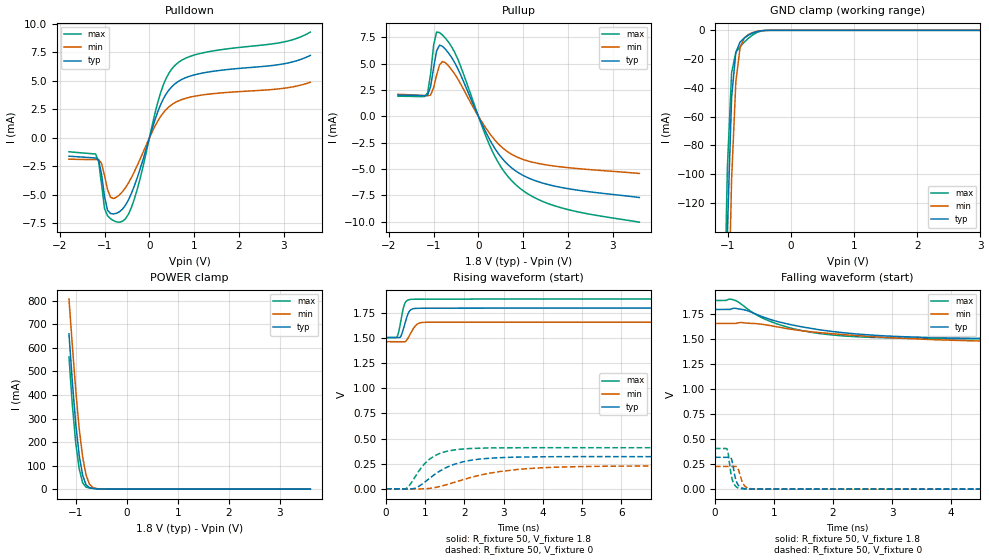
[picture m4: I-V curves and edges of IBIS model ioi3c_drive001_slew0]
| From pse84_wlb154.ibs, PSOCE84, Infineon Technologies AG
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[Model] ioi3c_drive001_slew0
Model_type I/O
Enable   Active-High
Vinl  =  0.54
Vinh  =  1.26
Vmeas =  0.9
Cref  =  15e-12
| Capacitance   typ   min   max
C_comp   9.12545e-13 8.87504e-13 9.42456e-13
| Variables   typ   min   max
[GND Clamp Reference]   0   0   0
[POWER Clamp Reference]   1.8   1.66   1.89
[Pulldown Reference]   0   0   0
[Pullup Reference]   1.8   1.66   1.89
[Temperature Range]   25   125   -40
[Voltage Range]   1.8   1.66   1.89
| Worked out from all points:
|   slope of the pulldown table from 0 to 0.27 V, typ, clamps not added: 87.9 ohm
|   slope of the pullup table from 0 to 0.27 V, typ, clamps not added: 115 ohm
|   GND clamp passes 1 mA (typ) near -0.55 V on its own axis
|   POWER clamp passes 1 mA (typ) near -0.54 V on its own axis
|   falling waveform, R_fixture 50, V_fixture 1.8: 20-80 % time 1.48ns typ, 2.34ns min, 990ps max; typ from 1.8 V to 1.51 V
|   falling waveform, R_fixture 50, V_fixture 0: 20-80 % time 73ps typ, 80.4ps min, 68.9ps max; typ from 0.319 V to 0 V
|   rising waveform, R_fixture 50, V_fixture 1.8: 20-80 % time 136ps typ, 178ps min, 116ps max; typ from 1.51 V to 1.8 V
|   rising waveform, R_fixture 50, V_fixture 0: 20-80 % time 866ps typ, 1.54ns min, 553ps max; typ from 0 V to 0.319 V
[GND Clamp]
| Voltage   I(typ)   I(min)   I(max)
-1.204V   -737.9mA   -831.5mA   -678.7mA
-1.07V    -303.2mA   -410.8mA   -239.8mA
-1.003V   -139.9mA   -232.2mA   -95.74mA
-936.6mV  -46.51mA   -103.5mA   -29.5mA
-869.7mV  -15.31mA   -35.88mA   -15.36mA
-802.8mV  -8.166mA   -12.13mA   -11.29mA
-735.9mV  -5.335mA   -5.292mA   -8.195mA
-669mV    -3.356mA   -2.85mA    -5.457mA
-535.2mV  -837.9uA   -772uA     -1.483mA
-401.4mV  -47.36uA   -84.85uA   -76.77uA
3.6V      0A         0A         0A
[POWER Clamp]
| Voltage   I(typ)   I(min)   I(max)
-1.137V   660mA      807.5mA    561.8mA
-1.07V    454.5mA    608.2mA    356.2mA
-1.003V   275.7mA    418.4mA    193.6mA
-936.6mV  143.5mA    257.2mA    86.91mA
-869.7mV  59.43mA    137.9mA    27.31mA
-802.8mV  18.8mA     60.93mA    8.704mA
-735.9mV  6.231mA    21.35mA    5.155mA
-669mV    3.127mA    6.887mA    3.44mA
-535.2mV  940.9uA    1.232mA    1.058mA
-334.5mV  16.1uA     59.03uA    7.686uA
3.6V      0A         0A         0A
[Pulldown]
| Voltage   I(typ)   I(min)   I(max)
-1.8V     -1.61mA    -1.871mA   -1.222mA
-1.204V   -1.765mA   -1.911mA   -1.417mA
-1.137V   -1.93mA    -1.912mA   -2.077mA
-1.003V   -5.181mA   -3.312mA   -6.214mA
-936.6mV  -6.363mA   -4.544mA   -6.839mA
-869.7mV  -6.641mA   -5.216mA   -7.096mA
-602.1mV  -6.249mA   -4.717mA   -7.32mA
-334.5mV  -4.187mA   -2.945mA   -5.335mA
248.3mV   2.889mA    1.862mA    3.936mA
558.6mV   4.697mA    3.058mA    6.305mA
1.117V    5.626mA    3.722mA    7.382mA
3.6V      7.233mA    4.878mA    9.276mA
[Pullup]
| Voltage   I(typ)   I(min)   I(max)
-1.8V     2.028mA    2.104mA    1.92mA
-1.137V   2.037mA    1.961mA    2.234mA
-1.07V    2.828mA    2.023mA    4.027mA
-1.003V   4.601mA    2.729mA    6.745mA
-936.6mV  6.228mA    3.912mA    8.012mA
-869.7mV  6.772mA    4.901mA    7.966mA
-735.9mV  6.371mA    5.088mA    7.421mA
-468.3mV  4.596mA    3.596mA    5.503mA
310.3mV   -2.648mA   -1.955mA   -3.309mA
806.9mV   -5.099mA   -3.749mA   -6.382mA
1.738V    -6.654mA   -4.742mA   -8.542mA
3.6V      -7.709mA   -5.424mA   -10.05mA
[Ramp]
dV/dt_r   0.19169/0.866128n  0.136435/1.54267n  0.244811/0.553181n
dV/dt_f   0.176398/1.47748n  0.116708/2.34317n  0.230254/0.990369n
R_load = 50
[Falling Waveform]
R_fixture = 50
V_fixture = 1.8
V_fixture_min = 1.66
V_fixture_max = 1.89
| Time   V(typ)   V(min)   V(max)
0s        1.8V       1.66V      1.89V
331.7ps   1.812V     1.66V      1.893V
563.3ps   1.786V     1.662V     1.8V
920.2ps   1.703V     1.641V     1.684V
1.322ns   1.643V     1.599V     1.608V
1.773ns   1.596V     1.568V     1.559V
2.883ns   1.535V     1.521V     1.516V
4.685ns   1.51V      1.481V     1.506V
10.33ns   1.505V     1.465V     1.506V
800ns     1.506V     1.465V     1.506V
[Falling Waveform]
R_fixture = 50
V_fixture = 0
V_fixture_min = 0
V_fixture_max = 0
| Time   V(typ)   V(min)   V(max)
0s        319.5mV    227.4mV    408mV
205ps     319.4mV    227.4mV    402.1mV
225.6ps   319.1mV    227.4mV    353mV
288.4ps   286.1mV    227.3mV    106.7mV
339.4ps   125.7mV    227.9mV    36.66mV
372.2ps   64.2mV     223.1mV    18.07mV
471.3ps   9.169mV    60.71mV    2.247mV
540.4ps   2.647mV    16.12mV    983.9uV
1.123ns   450.6uV    489.3uV    355.2uV
800ns     18.03nV    1.09uV     7.328nV
[Rising Waveform]
R_fixture = 50
V_fixture = 1.8
V_fixture_min = 1.66
V_fixture_max = 1.89
| Time   V(typ)   V(min)   V(max)
0s        1.506V     1.465V     1.506V
283.7ps   1.506V     1.465V     1.513V
329.1ps   1.505V     1.465V     1.569V
387.1ps   1.524V     1.466V     1.687V
467.5ps   1.623V     1.464V     1.832V
543.8ps   1.724V     1.488V     1.877V
639.1ps   1.785V     1.555V     1.887V
845.9ps   1.799V     1.651V     1.889V
1.684ns   1.8V       1.659V     1.89V
800ns     1.8V       1.66V      1.89V
[Rising Waveform]
R_fixture = 50
V_fixture = 0
V_fixture_min = 0
V_fixture_max = 0
| Time   V(typ)   V(min)   V(max)
0s        18.03nV    1.09uV     7.328nV
520.7ps   -3.108mV   -1.146mV   4.327mV
754.4ps   7.688mV    -2.095mV   125.4mV
966.3ps   58.38mV    -694.7uV   241.2mV
1.337ns   167mV      18.5mV     346.5mV
1.972ns   269.3mV    91.79mV    395.8mV
2.608ns   302.8mV    152.2mV    406.8mV
3.987ns   318.7mV    209.2mV    409mV
6.868ns   320.2mV    227.4mV    408.2mV
50ns      319.5mV    227.4mV    408mV
